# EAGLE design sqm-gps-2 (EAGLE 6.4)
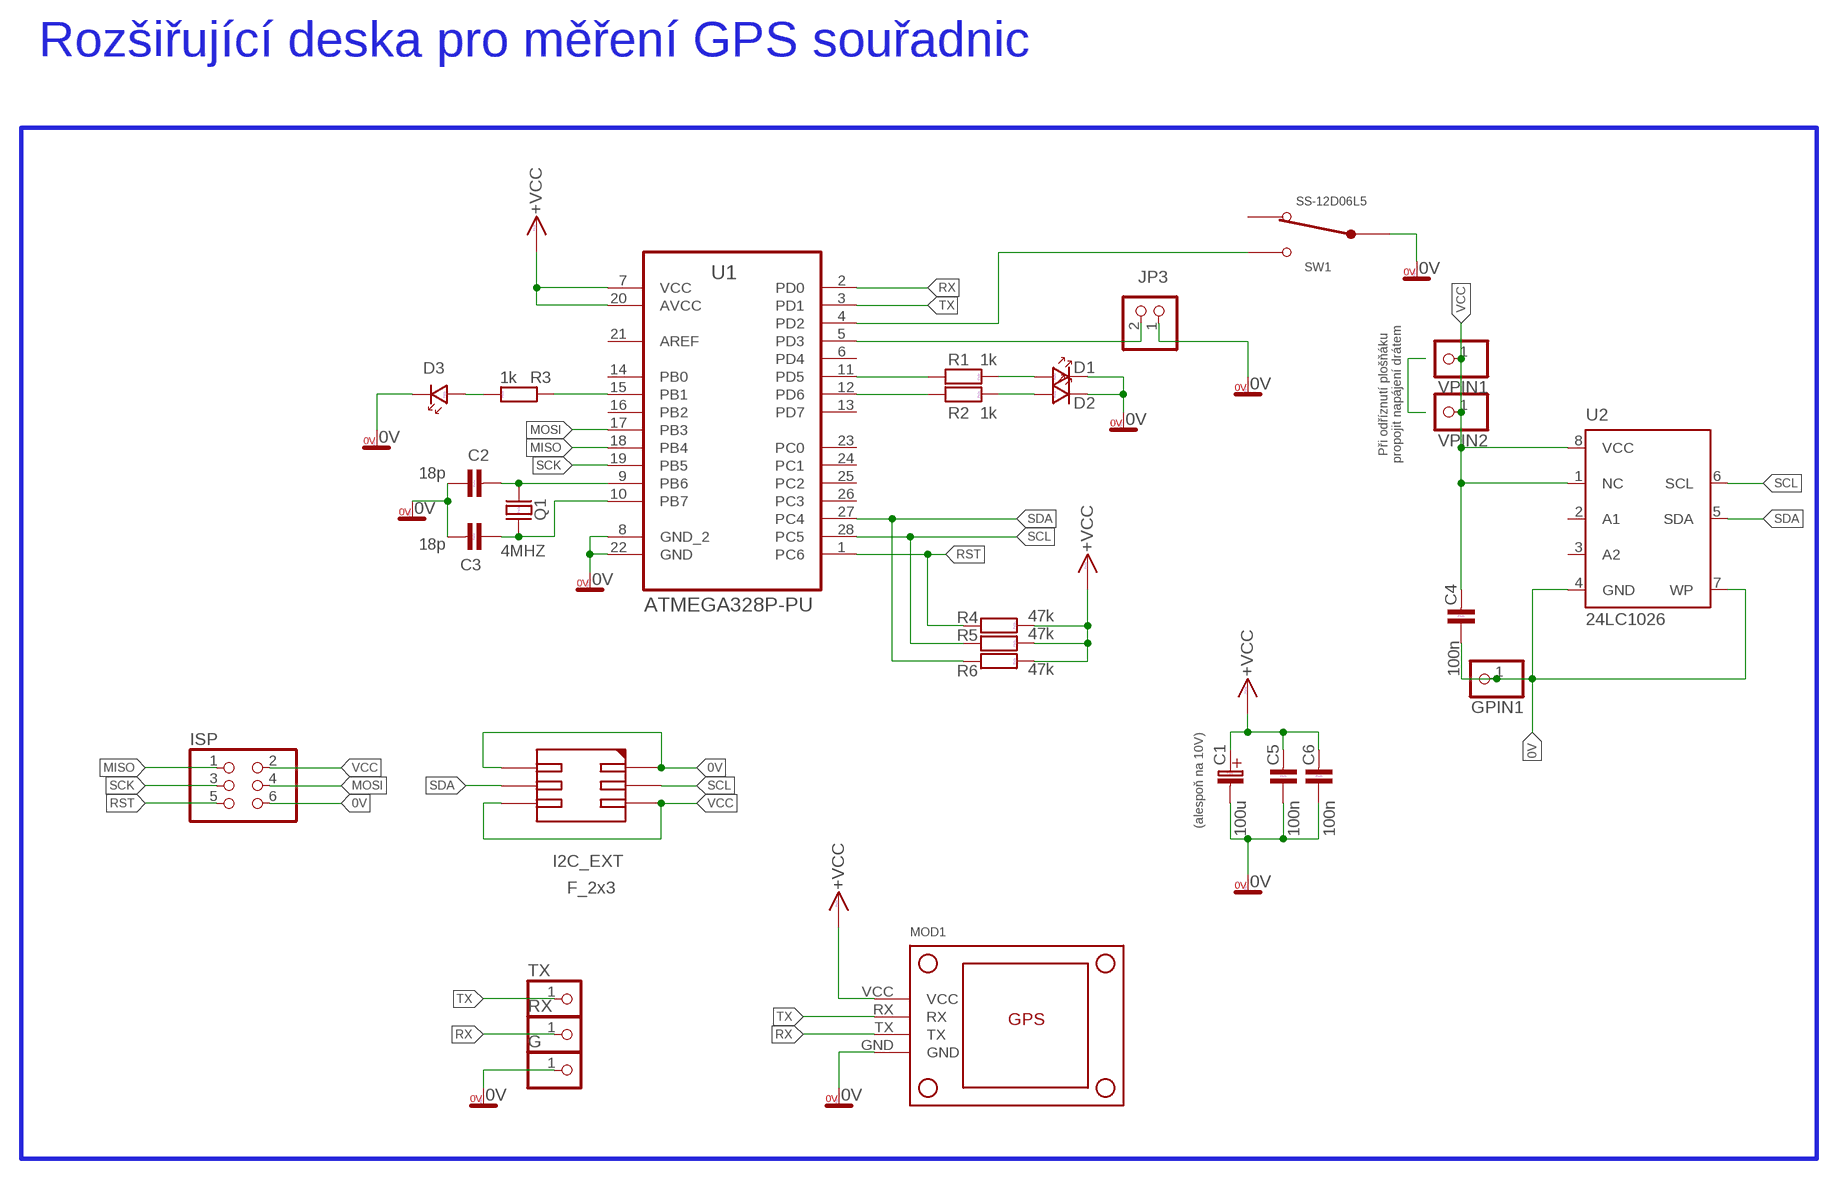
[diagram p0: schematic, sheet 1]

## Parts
C1  100u  C-ELEKTROLYT_3,5  [C-EL_3,5]
C2  18p  C-KERAMIK_SMD_0805  [0805]
C3  18p  C-KERAMIK_SMD_0805  [0805]
C4  100n  C-KERAMIK_SMD_0805  [0805]
C5  100n  C-KERAMIK_SMD_0805  [0805]
C6  100n  C-KERAMIK_SMD_0805  [0805]
D1  LED_3  [LED_3]
D2  LED_3  [LED_3]
D3  LED_3  [LED_3]
G  PINHD-1X1  [1X01]
GPIN1  PINHD-1X1  [1X01]
I2C_EXT  F_2x3  DUTINKY_2X3  [DUTINKY_2X3]
ISP  PINHD-2X3  [2X03]
JP3  PINHD-1X2/90  [1X02/90]
MOD1  GPS_MODUL  [GPS_MODUL]
Q1  4MHZ  Q_HC-49U  [HC-49U]
R1  1k  R_SMD_0805  [0805]
R2  1k  R_SMD_0805  [0805]
R3  1k  R_SMD_0805  [0805]
R4  47k  R_SMD_0805  [0805]
R5  47k  R_SMD_0805  [0805]
R6  47k  R_SMD_0805  [0805]
RX  PINHD-1X1  [1X01]
SW1  SS-12D06L5  SLIDE_SW  [SLIDE_SW]
TX  PINHD-1X1  [1X01]
U1  ATMEGA328P-PU  [DIP254P762X457-28]
U2  24LC1026  [SOIC8]
VPIN1  PINHD-1X1  [1X01]
VPIN2  PINHD-1X1  [1X01]

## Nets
0V: C1.C-(C_EL-) C2.1 C3.2 C4.1 C5.1 C6.1 D1.K D2.K D3.K G.1 GPIN1.1 I2C_EXT.PIN1 I2C_EXT.PIN2 ISP.6 JP3.1 MOD1.GND SW1.PIN_COM U1.8(GND_2) U1.22(GND) U2.4(GND) U2.7(WP)
B1: R3.1 U1.15(PB1)
B6: C2.2 Q1.2 U1.9(PB6)
B7: C3.1 Q1.1 U1.10(PB7)
D2: SW1.PIN_2 U1.4(PD2)
D3: JP3.2 U1.5(PD3)
D5: R1.1 U1.11(PD5)
D6: R2.1 U1.12(PD6)
LED1_A: D1.A R1.2
LED2_A: D2.A R2.2
LED3_A: D3.A R3.2
MISO: ISP.1 U1.18(PB4)
MOSI: ISP.4 U1.17(PB3)
RST: ISP.5 R4.1 U1.1(PC6)
RX: MOD1.TX RX.1 U1.2(PD0)
SCK: ISP.3 U1.19(PB5)
SCL: I2C_EXT.PIN3 R5.1 U1.28(PC5) U2.6(SCL)
SDA: I2C_EXT.PIN4 R6.1 U1.27(PC4) U2.5(SDA)
TX: MOD1.RX TX.1 U1.3(PD1)
VCC: C1.C+(C_EL+) C4.2 C5.2 C6.2 I2C_EXT.PIN5 I2C_EXT.PIN6 ISP.2 MOD1.VCC R4.2 R5.2 R6.2 U1.7(VCC) U1.20(AVCC) U2.1(NC) U2.8(VCC) VPIN1.1 VPIN2.1 ; supply symbol labelled +VCC
Unconnected: SW1.PIN_1 U1.6(PD4) U1.13(PD7) U1.14(PB0) U1.16(PB2) U1.21(AREF) U1.23(PC0) U1.24(PC1) U1.25(PC2) U1.26(PC3) U2.2(A1) U2.3(A2)

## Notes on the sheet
- Rozšiřující deska pro měření GPS souřadnic
- Při odříznutí plošňáku
  propojit napájení drátem
- (alespoň na 10V)

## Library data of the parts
C1 = #PaJa_30:C-ELEKTROLYT: Kondenzator - elektrolyticky
C2-C6 = #PaJa_30:C-KERAMIK: Kondenzator - keramicky
D1-D3 = #PaJa_30:LED: LED - jednobarevna
G GPIN1 RX TX VPIN1 VPIN2 = pinhead:PINHD-1X1: PIN HEADER
I2C_EXT = dutinky_2x3:DUTINKY_2X3
ISP = pinhead:PINHD-2X3: PIN HEADER
JP3 = pinhead:PINHD-1X2: PIN HEADER
MOD1 = GPS_MODUL:GPS_MODUL: GPS modul
Q1 = #PaJa_30:Q_HC-49U: Krystal - 1MHz - 48MHz
R1-R6 = #PaJa_30:R: Rezistor
SW1 = SLIDE_SW:SLIDE_SW: Posuvny prepinac
U1 = Atmel_By_element14_Batch_1-00:ATMEGA328P-PU: 8-bit Microcontroller with In-System Programmable Flash; MPN: ATMEGA328P-PU; OC_FARNELL: 1715487; OC_NEWARK: 15R0268; PACKAGE: PDIP-28; SUPPLIER: Atmel
U2 = 24lc1026:24LC1026: EEPROM - I2C 128k x 8b

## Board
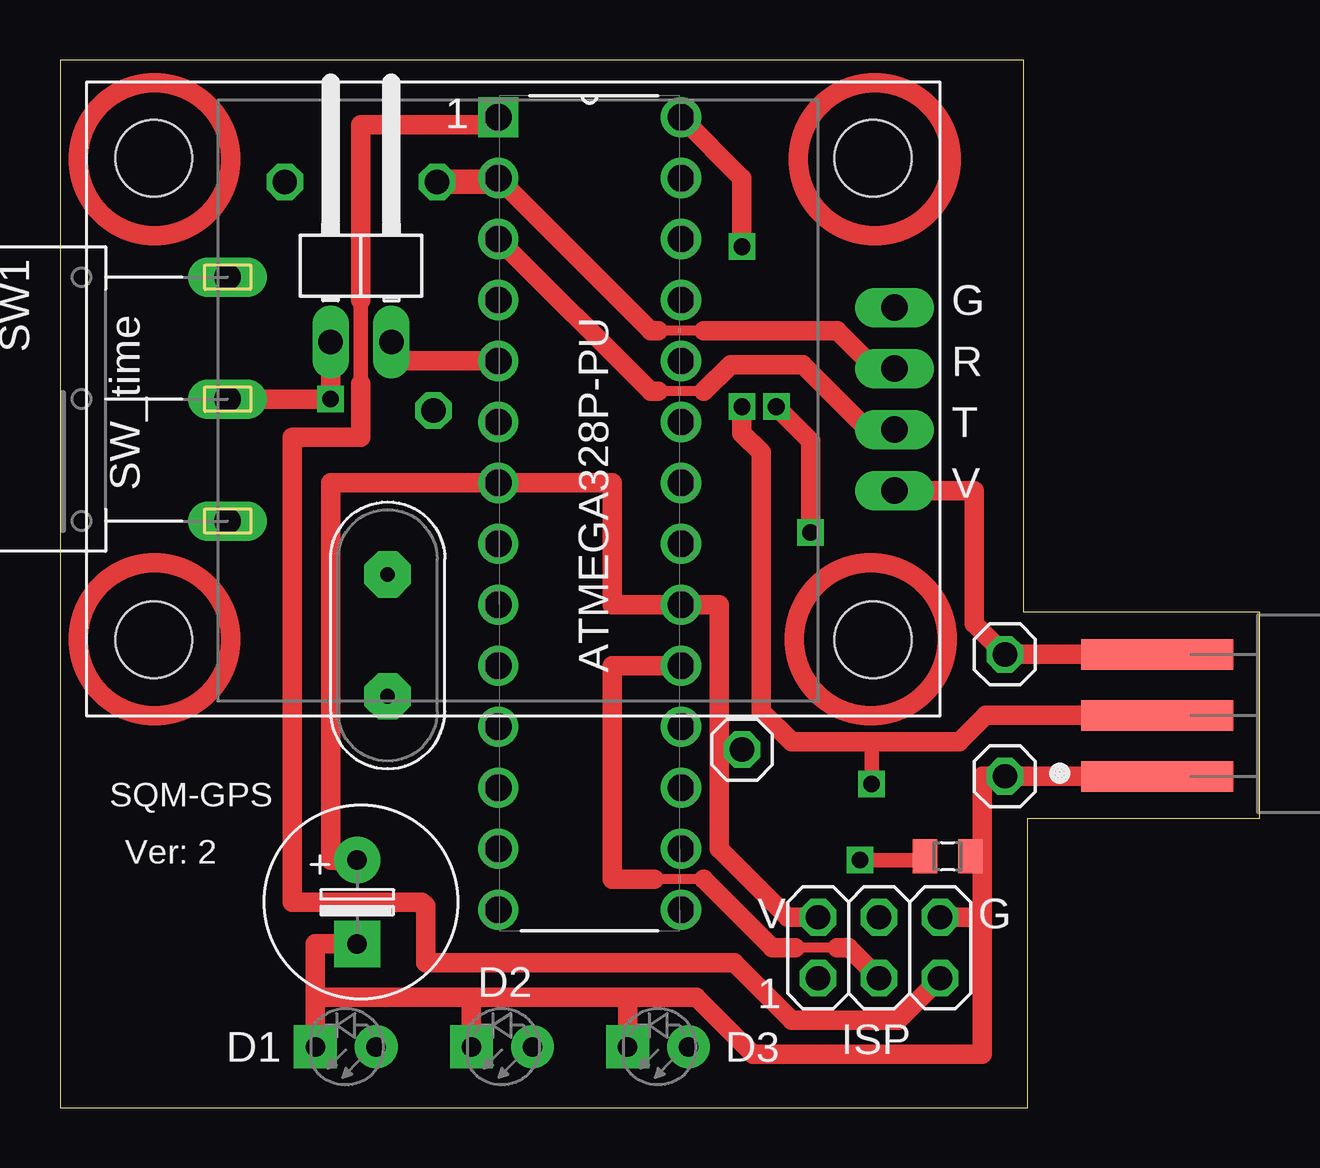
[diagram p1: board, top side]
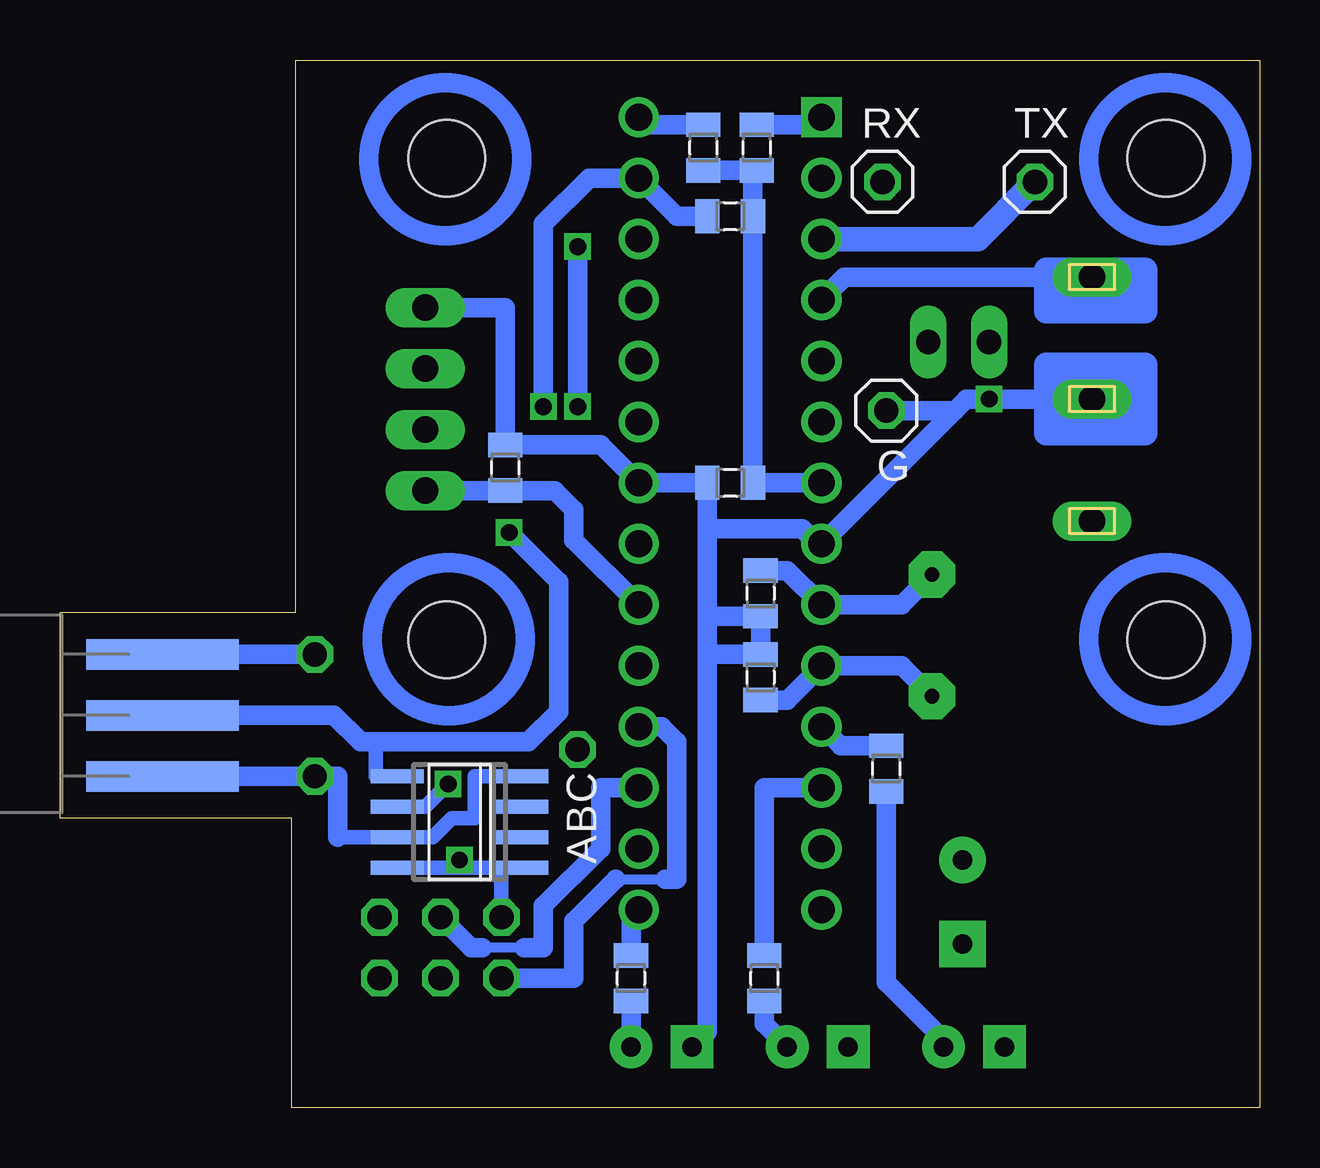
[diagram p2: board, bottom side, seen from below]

Size 49.99 x 43.66 mm. Coordinates in mm from the lower left corner, seen from the top.
Outline: 0,0 40.32,0 40.32,12.06 49.99,12.06 49.99,20.64 40.16,20.64 40.16,43.66 0,43.66 0,0
Copper layers (1*16): Top 0.035mm / dielectric 1.5mm / Bottom 0.035mm
Design rules "default *": minimum track width 10mil, minimum drill 24mil, track to track 8mil, track to pad 8mil, pad to pad 8mil, via to via 8mil, smd to smd 8mil, copper to edge 40mil, drill to drill 8mil, minimum pad ring 10mil, minimum via ring 8mil, stop-mask expansion 4mil, vias tented up to drill 0mil, thermal gap 10mil

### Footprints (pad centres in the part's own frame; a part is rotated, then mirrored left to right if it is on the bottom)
C-EL_3,5 = drill 0.813 pad 1.93: C+ 0,0 | drill 0.813 pad 1.93 square: C- 3.493,0
0805 = smd 1.016 x 1.422: 1 -0.953,0; 2 0.953,0
LED_3 = drill 0.813 pad 1.778: A -1.27,0 | drill 0.813 pad 1.778 square: K 1.27,0
1X01 = drill 1.016 octagon: 1 0,0
DUTINKY_2X3 = smd 6.35 x 1.27: PIN1 0,-2.54; PIN3 0,0; PIN5 0,2.54 | smd 6.35 x 1.27 bottom: PIN2 0,-2.54; PIN4 0,0; PIN6 0,2.54
2X03 = drill 1.016 octagon: 1 -2.54,-1.27; 2 -2.54,1.27; 3 0,-1.27; 4 0,1.27; 5 2.54,-1.27; 6 2.54,1.27
1X02/90 = drill 1.016 long: 1 -1.27,-3.81; 2 1.27,-3.81
GPS_MODUL = drill 1.1 long: GND 3.81,0; RX -1.27,0; TX 1.27,0; VCC -3.81,0 | hole 3.2: -10.033,0.889; 10.033,0.889; 10.033,30.861; -10.033,30.861
HC-49U = drill 0.61 pad 1.93 octagon: 1 -2.54,0; 2 2.54,0
SLIDE_SW = drill 1.1 long: PIN_1 -5.08,-7.62; PIN_2 5.08,-7.62; PIN_COM 0,-7.62
DIP254P762X457-28 = drill 1.118 square: 1 -7.62,33.02 | drill 1.118: 2 -7.62,30.48; 3 -7.62,27.94; 4 -7.62,25.4; 5 -7.62,22.86; 6 -7.62,20.32; 7 -7.62,17.78; 8 -7.62,15.24; 9 -7.62,12.7; 10 -7.62,10.16; 11 -7.62,7.62; 12 -7.62,5.08; 13 -7.62,2.54; 14 -7.62,0; 15 0,0; 16 0,2.54; 17 0,5.08; 18 0,7.62; 19 0,10.16; 20 0,12.7; 21 0,15.24; 22 0,17.78; 23 0,20.32; 24 0,22.86; 25 0,25.4; 26 0,27.94; 27 0,30.48; 28 0,33.02
SOIC8 = smd 0.6 x 2.2: 1 -1.905,-2.6; 2 -0.635,-2.6; 3 0.635,-2.6; 4 1.905,-2.6; 5 1.905,2.6; 6 0.635,2.6; 7 -0.635,2.6; 8 -1.905,2.6

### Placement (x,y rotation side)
C1  12.38,10.32 270 top
C2  20.8,21.43 90 bottom
C3  20.8,17.94 90 bottom
C4  36.99,10.48 180 top
C5  22.07,26.04 0 bottom
C6  31.43,26.67 270 bottom
D1  11.91,2.54 180 top
D2  18.41,2.54 180 top
D3  24.92,2.54 180 top
G  15.56,29.05 0 bottom
GPIN1  39.37,13.81 0 top
I2C_EXT  45.72,16.35 0 top
ISP  34.13,6.67 0 top
JP3  12.54,35.72 0 top
MOD1  34.77,29.53 90 top
Q1  13.65,19.68 90 top
R1  15.56,14.13 270 bottom
R2  20.64,5.4 270 bottom
R3  26.19,5.4 270 bottom
R4  20.95,40.01 270 bottom
R5  23.18,40.01 270 bottom
R6  22.07,37.15 0 bottom
RX  15.72,38.58 0 bottom
SW1  -0.64,29.53 90 top
TX  9.37,38.58 0 bottom
U1  25.88,8.26 0 top
U2  33.34,11.91 90 bottom
VPIN1  28.42,14.92 0 top
VPIN2  39.37,18.89 0 top

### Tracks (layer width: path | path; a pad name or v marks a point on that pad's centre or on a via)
0V  (via drill 0.7)
  Top 0.61: C4.1 38.42,10.48 38.42,7.3
  Top 0.813: JP3.1 v11.27,29.53 SW1.PIN_COM | D1.K 10.64,4.6 | 10.64,4.6 10.64,6.83 C1.C- | D2.K 17.14,4.6 | 17.14,4.6 10.64,4.6 | 17.14,4.6 23.65,4.6 | 23.65,4.6 26.51,4.6 28.89,2.22 38.42,2.22 38.42,7.3 38.42,7.94 | 38.42,7.94 ISP.6 | 23.65,4.6 D3.K | 38.42,7.94 38.42,13.81 GPIN1.1 I2C_EXT.PIN2
  Bottom 0.61: 38.42,11.27 U2.7 34.45,11.27 33.66,12.06 32.7,12.06 32.7,13.81 U2.4
  Bottom 0.813: 12.7,29.05 U1.8 18.41,23.5 19.05,24.13 23.02,24.13 | MOD1.GND 31.43,33.34 C6.1 27.46,27.62 U1.22 C5.1 23.02,24.13 | 23.02,20.48 C2.1 C3.2 23.02,18.89 | 23.02,20.48 23.02,24.13 | D3.K 23.02,3.17 23.02,18.89 | 23.02,18.89 23.02,20.48 | 45.88,13.81 I2C_EXT.PIN2 GPIN1.1 38.42,13.81 38.42,11.27 | SW1.PIN_COM v11.27,29.53 12.22,29.53 12.7,29.05 | G.1 12.7,29.05
  Bottom 1.016: SW1.PIN_COM 6.99,30.96 | 6.99,30.96 5.56,30.96 | 5.56,30.96 4.76,30.96 4.76,28.1 8.89,28.1 8.89,30.96 6.99,30.96 | 5.56,30.96 5.56,28.89 8.26,28.89 8.26,30.16 6.03,30.16 6.03,28.26 6.35,28.26
B1
  Bottom 0.813: R3.1 26.19,8.26 U1.15
B6
  Bottom 0.813: Q1.2 14.92,20.95 U1.9 19.68,22.38 C2.2
B7
  Bottom 0.813: Q1.1 14.92,18.41 U1.10 19.68,16.99 C3.1
D2
  Bottom 0.813: U1.4 17.3,34.61 SW1.PIN_2
  Bottom 1.016: SW1.PIN_2 6.99,33.18 | 6.99,33.18 8.89,33.18 8.89,34.13 | 8.89,34.13 8.89,34.77 8.89,34.92 4.76,34.92 4.76,34.13 8.89,34.13 | 6.99,33.18 4.76,33.18 4.76,34.77
D3
  Top 0.813: JP3.2 13.81,31.11 U1.5
D5
  Bottom 0.813: R1.1 17.46,15.08 U1.11
D6
  Bottom 0.813: U1.12 20.64,13.34 R2.1
LED1_A
  Bottom 0.813: D1.A 13.18,2.86 15.56,5.24 R1.2
LED2_A
  Bottom 0.813: D2.A 20.64,3.49 R2.2
LED3_A
  Bottom 0.813: D3.A R3.2
MISO
  Bottom 0.406: 26.83,9.53 24.77,9.53
  Bottom 0.813: ISP.1 28.57,5.4 28.57,7.78 26.83,9.53 | 24.77,9.53 24.29,9.53 24.29,15.24 24.92,15.88 U1.18
MOSI
  Bottom 0.406: 30.64,6.67 32.38,6.67
  Bottom 0.813: U1.17 27.46,13.34 27.46,10.79 29.84,8.41 29.84,6.67 30.64,6.67 | 32.38,6.67 32.86,6.67 ISP.4
RST
  Top 0.61: 12.54,30.16 12.54,33.66
  Top 0.813: ISP.5 34.92,3.65 30.48,3.65 28.1,6.03 15.24,6.03 15.24,8.41 15.08,8.57 9.68,8.57 9.68,27.94 12.54,27.94 12.54,30.16 | 12.54,33.66 12.54,40.96 18.26,40.96 U1.1
  Bottom 0.813: R4.1 18.57,40.96 U1.1
RX
  Top 0.406: 26.83,32.38 24.92,32.38
  Top 0.813: 26.83,32.38 32.38,32.38 33.97,30.8 MOD1.TX | 24.92,32.38 24.61,32.38 U1.2
  Top 1.016: U1.2 18.26,38.58 RX.1
SCK
  Top 0.406: 32.38,6.67 30.64,6.67 | 26.83,9.53 24.77,9.53
  Top 0.813: ISP.3 32.86,6.67 32.38,6.67 | 30.64,6.67 29.69,6.67 26.83,9.53 | 24.77,9.53 23.02,9.53 23.02,18.41 U1.19
SCL  (via drill 0.7)
  Top 0.61: v33.81,13.49 33.81,15.24 33.97,15.24
  Top 0.813: I2C_EXT.PIN3 38.58,16.35 37.47,15.24 33.97,15.24 30.48,15.24 29.21,16.51 29.21,27.3 28.42,28.1 v28.42,29.21 | v28.42,35.88 28.42,38.73 U1.28
  Bottom 0.61: U2.6 34.77,12.54 v33.81,13.49
  Bottom 0.813: R5.1 25.56,40.96 U1.28 | v28.42,29.21 v28.42,35.88
SDA  (via drill 0.7)
  Top 0.813: v31.27,23.97 31.27,27.78 v29.84,29.21
  Bottom 0.61: U2.5 36.83,13.81 36.83,15.24
  Bottom 0.813: R6.1 24.29,37.15 U1.27 27.94,38.73 29.84,36.83 v29.84,29.21 | I2C_EXT.PIN4 38.58,16.35 37.47,15.24 36.83,15.24 30.48,15.24 29.21,16.51 29.21,21.91 v31.27,23.97
TX
  Top 0.406: 26.83,29.84 24.92,29.84
  Top 0.813: 26.83,29.84 27.94,30.96 30.96,30.96 33.66,28.26 MOD1.RX | 24.92,29.84 24.61,29.84 U1.3
  Bottom 1.016: U1.3 11.75,36.2 TX.1
VCC  (via drill 0.7)
  Top 0.61: 27.46,14.76 27.46,14.92 VPIN1.1 | C4.2 36.04,10.32 v33.34,10.32
  Top 0.813: C1.C+ 11.27,10.32 11.27,26.04 U1.7 23.02,26.04 23.02,20.95 U1.20 27.46,20.95 27.46,14.92 27.46,10.79 30.32,7.94 ISP.2 | I2C_EXT.PIN6 VPIN2.1 38.1,20.16 38.1,25.72 MOD1.VCC
  Bottom 0.61: 33.34,10 U2.8 | U2.1 31.59,10 | 33.34,10 v33.34,10.32 | ISP.2 31.59,10 | 31.59,10 33.34,10
  Bottom 0.813: U1.7 C5.2 R6.2 21.11,39.05 R4.2 R5.2 | MOD1.VCC C6.2 29.37,25.72 28.57,24.92 28.57,23.65 U1.20 | 45.72,18.73 I2C_EXT.PIN6 VPIN2.1
(copper drawn outside any net)
  shapes: Bottom circle x4, Top circle x4

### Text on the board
tPlace: 1 | G | R | T | SW_time | V | SQM-GPS | Ver: 2 | V | G | 1
bPlace: C | B | A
